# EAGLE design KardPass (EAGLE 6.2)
Assembly variants: build
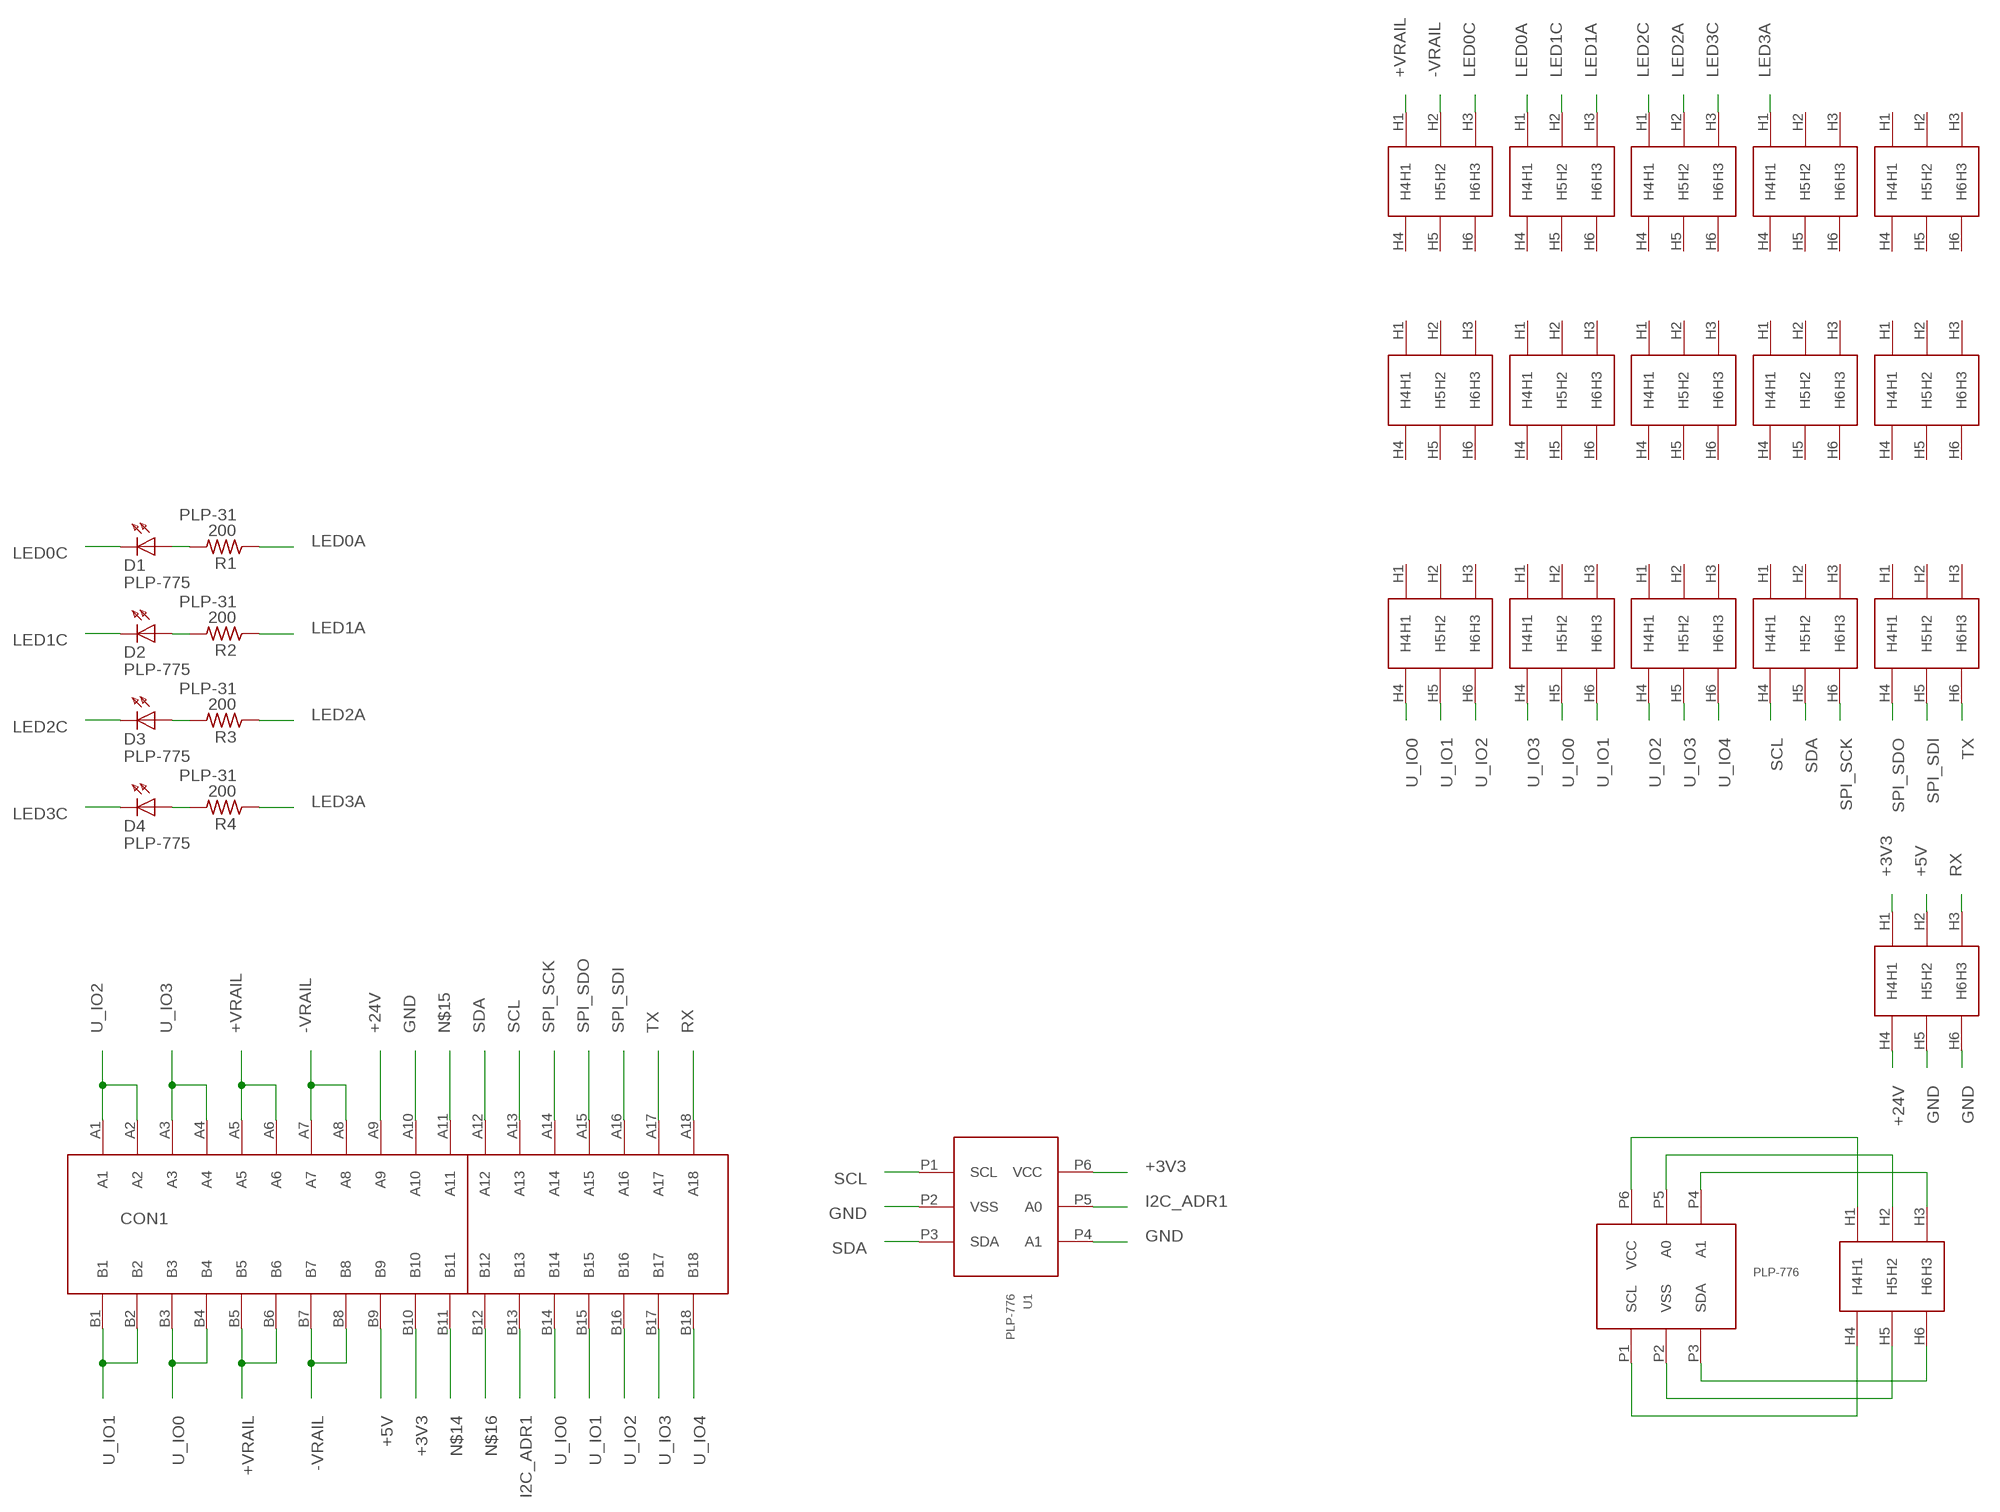
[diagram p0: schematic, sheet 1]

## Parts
CON1  PLPA-0107  [PLPA-0107]
D1  PLP-775  [PLP-775]
D2  PLP-775  [PLP-775]
D3  PLP-775  [PLP-775]
D4  PLP-775  [PLP-775]
H1  6HOLES  [6HOLES]  (not fitted in variant build)
H2  6HOLES  [6HOLES]  (not fitted in variant build)
H3  6HOLES  [6HOLES]  (not fitted in variant build)
H4  6HOLES  [6HOLES]  (not fitted in variant build)
H5  6HOLES  [6HOLES]  (not fitted in variant build)
H6  6HOLES  [6HOLES]  (not fitted in variant build)
H7  6HOLES  [6HOLES]  (not fitted in variant build)
H8  6HOLES  [6HOLES]  (not fitted in variant build)
H9  6HOLES  [6HOLES]  (not fitted in variant build)
H10  6HOLES  [6HOLES]  (not fitted in variant build)
H11  6HOLES  [6HOLES]  (not fitted in variant build)
H12  6HOLES  [6HOLES]  (not fitted in variant build)
H13  6HOLES  [6HOLES]  (not fitted in variant build)
H14  6HOLES  [6HOLES]  (not fitted in variant build)
H15  6HOLES  [6HOLES]  (not fitted in variant build)
H16  6HOLES  [6HOLES]  (not fitted in variant build)
H17  6HOLES  [6HOLES]  (not fitted in variant build)
R1  200  PLP-31  [DISCRETE_R0603]
R2  200  PLP-31  [DISCRETE_R0603]
R3  200  PLP-31  [DISCRETE_R0603]
R4  200  PLP-31  [DISCRETE_R0603]
U1  PLP-776  [SOT23-6]
   PLP-776  [SOT23-6]  (not fitted in variant build)

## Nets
+3V3: CON1.B10 H16.H1 U1.P6(VCC)
+5V: CON1.B9 H16.H2
+24V: CON1.A9 H16.H4
+VRAIL: CON1.A5 CON1.A6 CON1.B5 CON1.B6 H1.H1
-VRAIL: CON1.A7 CON1.A8 CON1.B7 CON1.B8 H1.H2
GND: CON1.A10 H16.H5 H16.H6 U1.P2(VSS) U1.P4(A1)
I2C_ADR1: CON1.B13 U1.P5(A0)
LED0A: H2.H1 R1.1
LED0C: D1.C H1.H3
LED1A: H2.H3 R2.1
LED1C: D2.C H2.H2
LED2A: H3.H2 R3.1
LED2C: D3.C H3.H1
LED3A: H4.H1 R4.1
LED3C: D4.C H3.H3
N$1: D1.A R1.2
N$2: D2.A R2.2
N$3: D3.A R3.2
N$4: D4.A R4.2
N$8: H17.H6  .P3(SDA)
N$9: H17.H5  .P2(VSS)
N$10: H17.H4  .P1(SCL)
N$11: H17.H3  .P4(A1)
N$12: H17.H2  .P5(A0)
N$13: H17.H1  .P6(VCC)
N$14: CON1.B11
N$15: CON1.A11
N$16: CON1.B12
RX: CON1.A18 H16.H3
SCL: CON1.A13 H14.H4 U1.P1(SCL)
SDA: CON1.A12 H14.H5 U1.P3(SDA)
SPI_SCK: CON1.A14 H14.H6
SPI_SDI: CON1.A16 H15.H5
SPI_SDO: CON1.A15 H15.H4
TX: CON1.A17 H15.H6
U_IO0: CON1.B3 CON1.B4 CON1.B14 H11.H4 H12.H5
U_IO1: CON1.B1 CON1.B2 CON1.B15 H11.H5 H12.H6
U_IO2: CON1.A1 CON1.A2 CON1.B16 H11.H6 H13.H4
U_IO3: CON1.A3 CON1.A4 CON1.B17 H12.H4 H13.H5
U_IO4: CON1.B18 H13.H6
Unconnected: H1.H4 H1.H5 H1.H6 H2.H4 H2.H5 H2.H6 H3.H4 H3.H5 H3.H6 H4.H2 H4.H3 H4.H4 H4.H5 H4.H6 H5.H1 H5.H2 H5.H3 H5.H4 H5.H5 H5.H6 H6.H1 H6.H2 H6.H3 H6.H4 H6.H5 H6.H6 H7.H1 H7.H2 H7.H3 H7.H4 H7.H5 H7.H6 H8.H1 H8.H2 H8.H3 H8.H4 H8.H5 H8.H6 H9.H1 H9.H2 H9.H3 H9.H4 H9.H5 H9.H6 H10.H1 H10.H2 H10.H3 H10.H4 H10.H5 H10.H6 H11.H1 H11.H2 H11.H3 H12.H1 H12.H2 H12.H3 H13.H1 H13.H2 H13.H3 H14.H1 H14.H2 H14.H3 H15.H1 H15.H2 H15.H3

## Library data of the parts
CON1 = PLP:PLPA-0107: CONN PCI EXPRESS 36POS VERT PCB; PLP#: PLPA-0107
D1-D4 = PLP:PLP-775: LED Green RT Ang; PLP#: PLP-775
H1-H17 = ms:6HOLES; PLP#: PLP-0
R1-R4 = PLP:PLP-31: Resistor; PLP#: PLP-31
U1   = PLP:PLP-776: IC EEPROM 2KBIT 400KHZ SOT23-6; PLP#: PLP-776

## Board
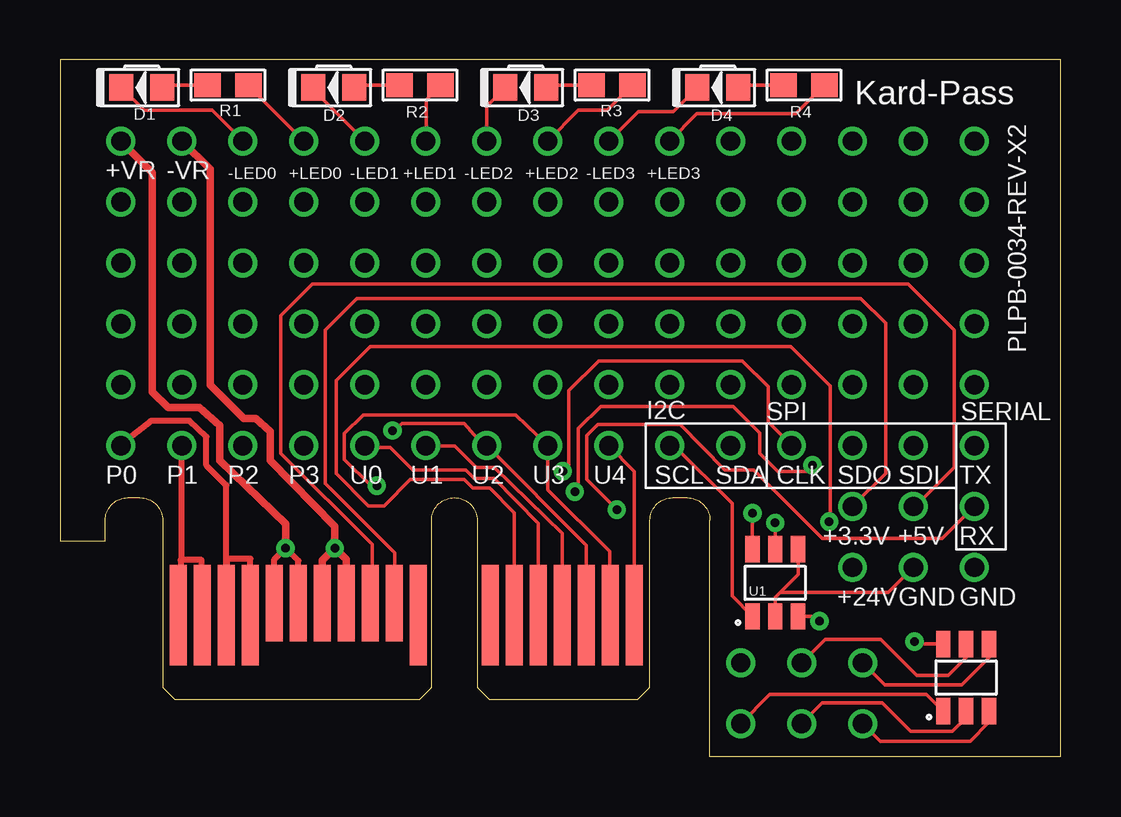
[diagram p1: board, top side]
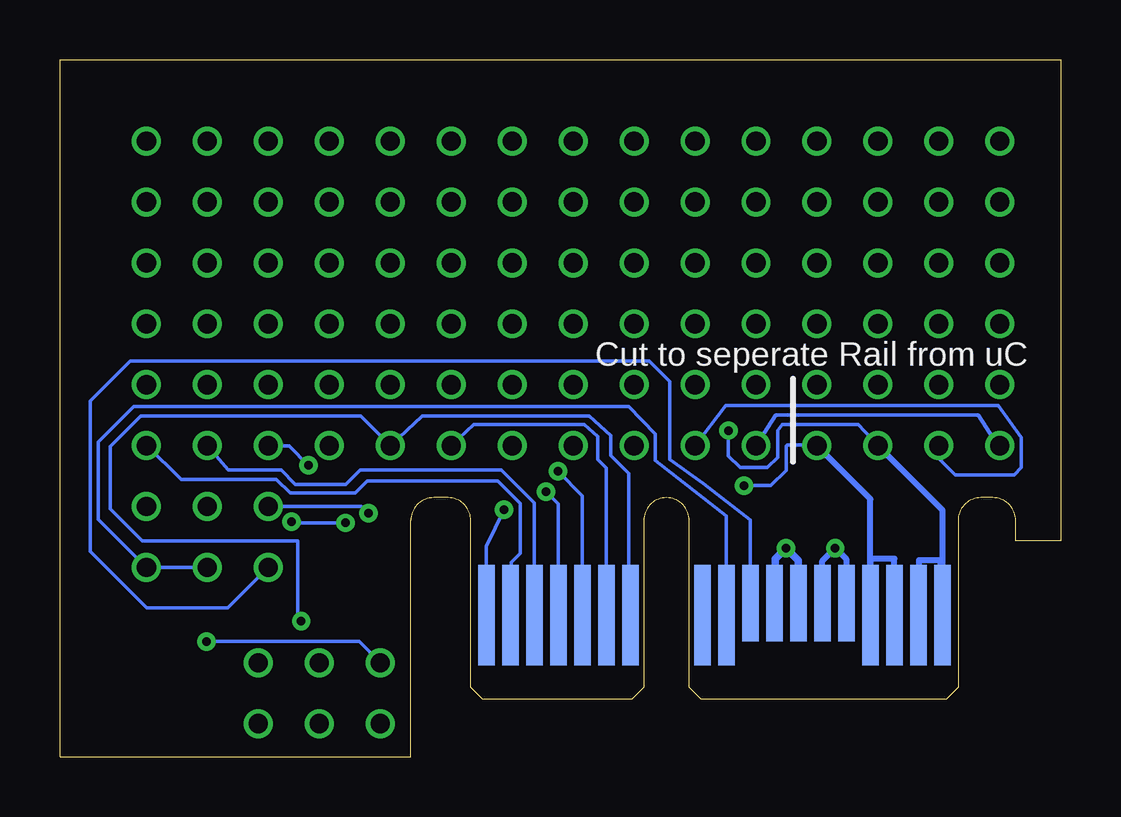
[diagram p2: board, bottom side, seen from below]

Size 41.7 x 29.05 mm. Coordinates in mm from the lower left corner, seen from the top.
Outline: 1.88,9.85 1.88,9 0,9 0,29.05 41.7,29.05 41.7,0 27.08,0 27.08,9.85
Copper layers (1*16): Top 0.0178mm / dielectric 59mil / Bottom 0.0178mm
Design rules: minimum track width 6mil, minimum drill 14mil, track to track 6mil, track to pad 6mil, pad to pad 6mil, via to via 6mil, smd to smd 6mil, copper to edge 20mil, drill to drill 16mil, minimum pad ring 8mil, minimum via ring 8mil, stop-mask expansion 3mil, vias tented up to drill 14mil, thermal gap 10mil
tKeepout: area 0,-1 to 0.8,29.1; area 41,-1 to 41.7,29.1
bKeepout: area 0,-1 to 0.8,29.1; area 41,-1 to 41.7,29.1

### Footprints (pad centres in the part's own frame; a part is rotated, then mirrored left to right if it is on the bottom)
PLPA-0107 = smd 0.7 x 4.2 bottom: A1 -11.5,3.5; A2 -10.5,3.5; A3 -9.5,3.5; A4 -8.5,3.5; A10 -2.5,3.5; A11 -1.5,3.5; A12 1.5,3.5; A13 2.5,3.5; A14 3.5,3.5; A15 4.5,3.5; A16 5.5,3.5; A17 6.5,3.5; A18 7.5,3.5 | smd 0.7 x 3.2 bottom: A5 -7.5,4; A6 -6.5,4; A7 -5.5,4; A8 -4.5,4; A9 -3.5,4 | smd 0.7 x 4.2: B1 -11.5,3.5; B2 -10.5,3.5; B3 -9.5,3.5; B4 -8.5,3.5; B11 -1.5,3.5; B12 1.5,3.5; B13 2.5,3.5; B14 3.5,3.5; B15 4.5,3.5; B16 5.5,3.5; B17 6.5,3.5; B18 7.5,3.5 | smd 0.7 x 3.2: B5 -7.5,4; B6 -6.5,4; B7 -5.5,4; B8 -4.5,4; B9 -3.5,4; B10 -2.5,4
PLP-775 = smd 1 x 1.1: A 0.85,0; C -0.85,0
6HOLES = drill 0.8: H1 -2.54,1.27; H2 0,1.27; H3 2.54,1.27; H4 -2.54,-1.27; H5 0,-1.27; H6 2.54,-1.27
DISCRETE_R0603 = smd 1.1 x 1: 1 -0.85,0; 2 0.85,0
SOT23-6 = smd 0.6 x 1.1: P1 -0.95,-1.4; P2 0,-1.4; P3 0.95,-1.4; P4 0.95,1.4; P5 0,1.4; P6 -0.95,1.4

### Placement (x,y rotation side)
CON1  16.43,2.4 0 top
D1  3.4,27.9 0 top
D2  11.4,27.9 0 top
D3  19.4,27.9 0 top
D4  27.4,27.9 0 top
H1  5.08,24.4 0 top
H2  12.7,24.4 0 top
H3  20.32,24.4 0 top
H4  27.94,24.4 0 top
H5  35.56,24.4 0 top
H6  5.08,19.32 0 top
H7  12.7,19.32 0 top
H8  20.32,19.32 0 top
H9  27.94,19.32 0 top
H10  35.56,19.32 0 top
H11  5.08,14.24 0 top
H12  12.7,14.24 0 top
H13  20.32,14.24 0 top
H14  27.94,14.24 0 top
H15  35.56,14.24 0 top
H16  35.56,9.16 0 top
H17  30.9,2.65 0 top
R1  7,28 180 top
R2  15,28 180 top
R3  23,28 180 top
R4  31,28 180 top
U1  29.8,7.25 0 top
   37.75,3.3 0 top

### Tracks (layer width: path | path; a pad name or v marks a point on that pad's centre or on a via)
+3V3  (via drill 0.36)
  Top 0.152: CON1.B10 13.95,5.92 13.95,8.5 11.05,11.4 11.05,17.78 12.37,19.1 33.37,19.1 34.4,18.07 34.4,11.81 H16.H1 | U1.P6 v28.85,10.15
  Bottom 0.152: v28.85,10.15 29.15,10.43 H16.H1
+5V
  Top 0.152: CON1.B9 13,5.97 13,8.85 9.2,12.65 9.2,18.39 10.51,19.7 35.34,19.7 37.25,17.79 37.25,12.05 35.63,10.43 H16.H2
+24V
  Bottom 0.152: CON1.A9 12.93,9.87 14.9,11.4 16.3,12.4 16.3,15.65 17.15,16.5 38.78,16.5 40.45,14.83 40.45,8.56 38.09,6.2 34.71,6.2 H16.H4
+VRAIL  (via drill 0.36)
  Top 0.254: CON1.A6 9.93,8.17 v9.4,8.7 8.93,8.23 CON1.A5
  Top 0.305: v9.4,8.7 9.4,9.7 6.65,12.35 6.65,13.8 5.8,14.55 4.5,14.55 3.85,15.2 3.85,24.35 H1.H1
  Bottom 0.254: CON1.A5 8.95,5.92 8.95,7.8 8.95,7.85 8.95,8.25 v9.4,8.7 9.93,8.17 CON1.A6
-VRAIL  (via drill 0.36)
  Top 0.305: CON1.A7 10.93,8.18 v11.45,8.7 | CON1.A8 11.93,8.22 v11.45,8.7 | v11.45,8.7 11.45,9.6 8.75,12.35 8.75,13.55 8.15,14.1 7.65,14.1 6.25,15.5 6.25,24.5 H1.H2
  Bottom 0.305: CON1.A8 11.93,6.82 11.9,6.85 11.9,8.25 v11.45,8.7 10.93,8.18 CON1.A7
GND
  Top 0.152: U1.P4 30.75,7.6 30,6.85 | 30,6.85 29.8,6.65 U1.P2 | H16.H5 34.52,6.85 30,6.85
  Bottom 0.152: CON1.A10 13.93,10.03 16.9,12.35 16.9,13.45 18,14.6 38.63,14.6 40.1,13.13 40.1,9.89 H16.H6 H16.H5
I2C_ADR1  (via drill 0.36)
  Top 0.152: CON1.B13 18.93,10.17 17.9,11.2 | 12.85,10.45 11.5,11.8 11.5,15.68 12.92,17.1 30.45,17.1 32.1,15.45 32.1,9.85 v32.05,9.8 | v29.8,9.75 U1.P5
  Top 0.155: 17.9,11.2 17.2,11.2 16.85,11.55 14.6,11.55 13.5,10.45 12.85,10.45
  Bottom 0.152: v32.05,9.8 32,9.75 v29.8,9.75
LED0A
  Top 0.152: R1.1 7.85,27.98 H2.H1
LED0C
  Top 0.152: D1.C 3.5,26.95 6.35,26.95 7.6,25.7 7.6,25.69 H1.H3
LED1A
  Top 0.152: R2.1 15.25,27.4 H2.H3
LED1C
  Top 0.152: D2.C 10.55,27.82 H2.H2
LED2A
  Top 0.152: R3.1 22.8,26.95 21.6,26.95 H3.H2
LED2C
  Top 0.152: D3.C 17.78,27.13 H3.H1
LED3A
  Top 0.152: R4.1 30.65,26.8 26.53,26.8 H4.H1
LED3C
  Top 0.152: D4.C 25.55,26.9 24.09,26.9 H3.H3
N$1
  Top 0.152: D1.A 4.35,28 R1.2
N$2
  Top 0.152: D2.A 12.35,28 R2.2
N$3
  Top 0.152: D3.A 20.35,28 R3.2
N$4
  Top 0.152: D4.A 28.35,28 R4.2
N$8
  Top 0.152: H17.H6 34.17,0.65 37.92,0.65 38.7,1.43  .P3
N$9
  Top 0.152: H17.H5 31.77,2.25 34.25,2.25 35.45,1.05 37.18,1.05 37.75,1.62  .P2
N$10
  Top 0.152: H17.H4 29.58,2.6 36.1,2.6  .P1
N$11
  Top 0.152: H17.H3 34.36,3 37.58,3 38.7,4.12  .P4
N$12
  Top 0.152: H17.H2 31.88,4.9 34.2,4.9 35.7,3.4 37,3.4 37.75,4.15 37.75,4.65 | 37.75,4.65 37.7,4.65 | 37.75,4.65  .P5
N$13  (via drill 0.36)
  Top 0.152: v35.6,4.8 35.7,4.7  .P6
  Bottom 0.152: H17.H1 29.24,4.8 v35.6,4.8
RX  (via drill 0.36)
  Top 0.152: H16.H3 36.77,9.1 31.75,9.1 28.9,11.95 27.7,11.95 25.85,13.85 22.41,13.85 21.95,13.39 21.95,12.35
  Top 0.155: 21.95,12.35 21.95,11.55 v23.2,10.3
  Bottom 0.152: CON1.A18 23.93,8.77 v23.2,10.3
SCL
  Top 0.152: H14.H4 25.58,12.97 28,10.55 28,6.7 U1.P1
  Bottom 0.152: CON1.A13 18.93,12.03 19.3,12.4 19.3,13.35 19.85,13.85 24.47,13.85 H14.H4
SDA  (via drill 0.36)
  Top 0.152: v31.65,5.65 31.45,5.85 U1.P3
  Bottom 0.152: 18.75,12.55 18.75,13.4 19.65,14.2 26.6,14.2 27.9,13 H14.H5 29.17,14.2 38.34,14.2 39.6,12.94 39.6,10.33 38.27,9 31.8,9 31.8,5.8 v31.65,5.65
  Bottom 0.155: 18.75,12.55 18,11.8 18,5.9 CON1.A12
SPI_SCK  (via drill 0.36)
  Top 0.152: v20.95,11.9 21.2,12.15 21.2,15.26 22.44,16.5 28.43,16.5 29.5,15.43 29.5,13.95 H14.H6
  Bottom 0.152: CON1.A14 19.93,10.88 v20.95,11.9
SPI_SDI
  Bottom 0.152: CON1.A16 21.93,10.57 23.31,11.95 29.2,11.95 29.8,11.35 31.89,11.35 32.49,11.95 34.7,11.95 H15.H5
SPI_SDO  (via drill 0.36)
  Top 0.152: v21.45,11.05 21.6,11.2 21.6,13.68 22.52,14.6 28.05,14.6 29.15,13.5 29.15,12.65 29.9,11.9 31.1,11.9 v31.35,12.15
  Bottom 0.152: CON1.A15 20.93,10.53 v21.45,11.05 | v31.35,12.15 32.15,12.95 33.05,12.95 H15.H4
TX
  Bottom 0.152: CON1.A17 22.9,8.1 22.53,8.47 22.53,10.56 23.47,11.5 28.9,11.5 29.4,11 32.1,11 32.7,11.55 36.65,11.55 38.1,13 H15.H6
U_IO0
  Top 0.152: CON1.B14 19.93,9.72 18.1,11.6 | 12.7,12.95 H12.H5 12.75,12.92 12.75,12.9
  Top 0.155: 12.75,12.9 13.75,12.9 14.7,11.95 16.9,11.95 17.25,11.6 18.1,11.6
  Top 0.254: CON1.B4 7.93,8.25 6.95,8.25 6.95,5.9 CON1.B3 6.93,11.32 6.1,12.15 6.1,13.35 5.4,14 3.8,14 2.6,13.05 H11.H4
  Bottom 0.152: H12.H5 11.87,14.25 3.45,14.25 2.62,12.97 H11.H4
U_IO1
  Top 0.152: CON1.B15 20.93,9.32 18.1,12.05
  Top 0.155: 18.1,12.05 17.35,12.05 16.45,12.95 15.25,12.95 H12.H6
  Top 0.254: CON1.B2 5.9,8.2 5.03,8.2 5.03,5.9 CON1.B1 | 5.05,5.9 CON1.B1 | CON1.B1 5.08,8.27 H11.H5
  Bottom 0.152: H12.H6 13.96,14.65 2.6,14.65 1.65,13.3 1.65,12.05 1.95,11.75 4.4,11.75 5.08,12.43 H11.H5
U_IO2  (via drill 0.36)
  Top 0.152: CON1.B16 21.93,8.82 17.8,12.95 | v13.85,13.6 14.25,13.9 16.85,13.9 17.65,12.95 17.8,12.95 | H13.H4 17.8,12.95
  Bottom 0.152: H11.H6 8.45,13.85 11.6,13.85 11.8,13.6 11.8,12.48 12.23,12.05 13.36,12.05 13.85,12.54 v13.85,13.6
  Bottom 0.254: CON1.A2 5.9,5.9 5.9,8.2 5.03,8.2 5.03,6.4 CON1.A1 4.93,10.28 H11.H6
U_IO3  (via drill 0.36)
  Top 0.152: v13.2,11.3 12.95,11.3 11.85,12.4 11.85,13.47 12.63,14.25 18.99,14.25 H13.H5
  Top 0.155: H13.H5 20.32,11.13 22.9,8.55 22.9,6.4 | 22.9,6.4 22.95,6.35 | CON1.B17 22.9,6.4
  Bottom 0.152: H12.H4 10.19,13 11.4,13 11.45,12.95 11.45,11.94 12.09,11.3 v13.2,11.3
  Bottom 0.254: H12.H4 7.93,10.74 CON1.A4 7.95,5.95 7.95,8.25 6.93,8.25 CON1.A3
U_IO4
  Top 0.152: CON1.B18 23.93,8.83
  Top 0.155: 23.93,8.83 23.93,11.9 H13.H6

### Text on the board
tPlace: Kard-Pass | +VR | -VR | -LED0 | +LED0 | -LED1 | +LED1 | -LED2 | +LED2 | -LED3 | +LED3 | PLPB-0034-REV-X2 | I2C | SPI | SERIAL | P0 | P1 | P2 | P3 | U0 | U1 | U2 | U3 | U4 | SCL | SDA | CLK | SDO | SDI | TX | +3.3V | +5V | RX | +24V | GND | GND
bPlace: Cut to seperate Rail from uC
